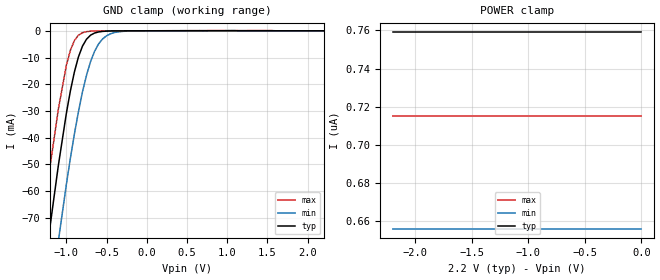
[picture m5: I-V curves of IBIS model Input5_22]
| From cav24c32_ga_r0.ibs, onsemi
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|//////////////////////////////////////////////////////////////////////////////
|//////////////////////////////////////////////////////////////////////////////
[Model]  Input5_22
Model_type Input
Vinh =  1.54
Vinl =  0.66
|  variable   typ   min   max
C_comp   6pF   NA   6pF
|//////////////////////////////////////////////////////////////////////////////
[Temperature Range]   25   NA   -40
|//////////////////////////////////////////////////////////////////////////////
[Voltage Range]   2.20V   NA   2.70V
|//////////////////////////////////////////////////////////////////////////////
[POWER Clamp Reference] 2.20V   NA   2.70V
|//////////////////////////////////////////////////////////////////////////////
[GND Clamp Reference]   0V   NA   0V
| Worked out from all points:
|   GND clamp passes 1 mA (typ) near -0.66 V on its own axis
|//////////////////////////////////////////////////////////////////////////////
[GND Clamp]
|   Voltage   I(typ)   I(min)   I(max)
-2.2V     -337mA     -365mA     -315mA
-1.3V     -96.4mA    -126mA     -73.6mA
-1.2V     -72.6mA    -102mA     -50.2mA
-1.1V     -50.5mA    -78.8mA    -29.4mA
-1V       -30.9mA    -57.5mA    -12.9mA
-950mV    -22.5mA    -47.7mA    -7.29mA
-850mV    -9.8mA     -30.3mA    -1.65mA
-800mV    -5.77mA    -22.9mA    -722uA
-650mV    -849uA     -7.73mA    -92.5uA
-550mV    -227uA     -3.07mA    -49.7uA
-400mV    -46.5uA    -651uA     -31.6uA
2.2V      759nA      656nA      715nA
|//////////////////////////////////////////////////////////////////////////////
[POWER Clamp]
|   Voltage   I(typ)   I(min)   I(max)
-2.2V     759nA      656nA      715nA
-2.1V     759nA      656nA      715nA
-2V       759nA      656nA      715nA
0V        759nA      656nA      715nA
